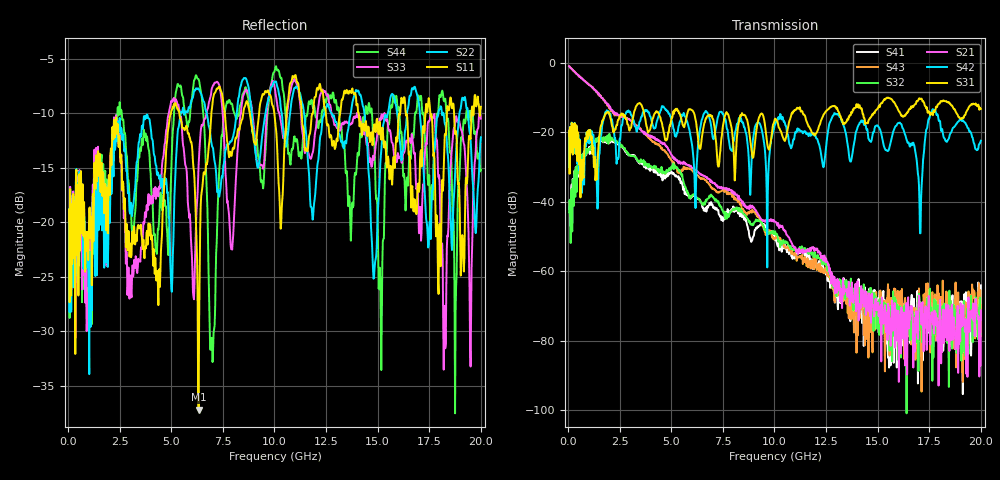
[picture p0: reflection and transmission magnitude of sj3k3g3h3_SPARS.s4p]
! FILE: E:\users\goganessyan\GBX_Backplane\FR408_backplane\1m_INBOUND_TRU\sj3k3g3h3_SPARS.s4p
# MHZ S RI R 50.00
! FREQ  S11  S12  S13  S14
!  S21  S22  S23  S24
!  S31  S32  S33  S34
!  S41  S42  S43  S44
!  REAL  IMAG  REAL  IMAG  REAL  IMAG  REAL  IMAG
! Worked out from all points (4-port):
!   799 points, 50 MHz to 20 GHz, reference 50 ohm
!   strongest paths, dB at 50 MHz, 5.025 GHz, 10.03 GHz, 15.03 GHz, 20 GHz:
!     S31: -19.6, -15.7, -16.1, -13.0, -13.3
!     S42: -19.6, -16.8, -17.8, -18.3, -22.5
!     S21: -1.0, -26.6, -45.8, -69.0, -71.3
!     S32: -43.1, -29.8, -48.6, -76.5, -78.1
!     S43: -1.1, -28.3, -50.4, -73.5, -78.7
!     S41: -42.1, -31.5, -51.1, -67.8, -64.1
!   lowest |S11| = -37.2 dB at 6.325 GHz (marker M1), VSWR 1.03, Z = 48.7 + j0.538 ohm
!   |S11| at or under -10 dB: start of sweep to 4.983 GHz; 5.391 GHz to 6.944 GHz (1.552 GHz wide, 25.2 % of centre); 14.08 GHz to 16.09 GHz (2.009 GHz wide, 13.3 % of centre)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
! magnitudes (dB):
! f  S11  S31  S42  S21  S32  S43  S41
! 50 MHz  -18.8  -19.6  -19.6  -1.0  -43.1  -1.1  -42.1
! 1.5 GHz  -15.0  -22.0  -26.6  -9.1  -21.5  -9.0  -21.2
! 6.325 GHz  -37.2  -23.4  -22.2  -31.7  -39.2  -32.7  -39.3
! 6.95 GHz  -9.8  -15.5  -19.1  -34.0  -38.3  -35.9  -40.5
! 10.03 GHz  -10.6  -16.1  -17.8  -45.8  -48.6  -50.4  -51.1
! 18.25 GHz  -12.0  -11.1  -21.9  -72.8  -72.4  -71.3  -70.8
! 20 GHz  -9.4  -13.3  -22.5  -71.3  -78.1  -78.7  -64.1
